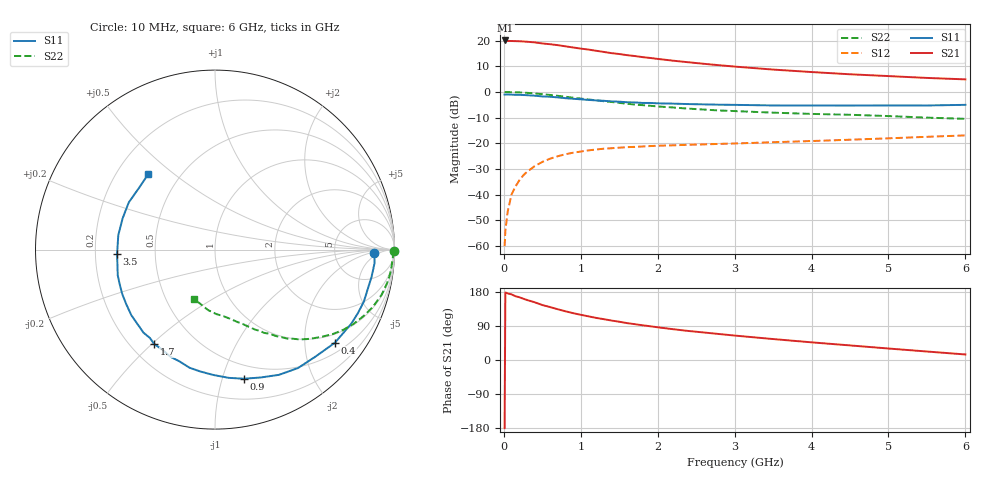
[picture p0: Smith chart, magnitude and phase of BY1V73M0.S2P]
! SIEMENS Small Signal Semiconductors
! BFY420
! Si NPN RF SIEGET Grounded Emitter Transistor in MICRO-X
! VCE = 1.75 V  IC = 3 mA
! Common Emitter S-Parameters:  October  1996
# GHz  S  MA  R  50
!  f  S11  S21  S12  S22
! GHz  MAG  ANG  MAG  ANG  MAG  ANG  MAG  ANG
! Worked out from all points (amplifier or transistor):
!   36 points, 10 MHz to 6 GHz, reference 50 ohm
!   highest |S21| = 20.0 dB at 20 MHz (marker M1)
!   |S21| within 3 dB of that: start of sweep to 962 MHz
!   unconditionally stable (mu >= 1): 3.603 GHz to end of sweep
!   at 250 MHz: K = 0.07, MSG = 26.1 dB, |S12| = -32.5 dB
!   at 1.4 GHz: K = 0.39, MSG = 18.5 dB, |S12| = -21.9 dB
!   at 6 GHz: K = 1.20, MAG = 8.2 dB, |S12| = -16.9 dB
!   S11 on the Smith chart (normalised r, x): 10 MHz: 16, -3; 400 MHz: 0.75, -2.74; 900 MHz: 0.37, -1.18; 1.7 GHz: 0.29, -0.51; 3.5 GHz: 0.29, -0.02; 6 GHz: 0.33, +0.41
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0.01  0.8887 -1.3  9.978 -179.8  0.001 111.1  0.9949 -0.5
0.02  0.8891 -2.0  10.04 178.2  0.002 96.4  0.992 -1.0
0.05  0.8923 -4.8  9.824 175.8  0.0047 90.2  0.9919 -2.5
0.1  0.8855 -9.8  9.789 173.1  0.0101 86.8  0.9884 -5.2
0.15  0.879 -14.4  9.742 168.4  0.0144 80.3  0.9851 -7.8
0.2  0.8785 -19.3  9.678 165.7  0.0189 79.5  0.9796 -10.2
0.3  0.8643 -28.5  9.48 158.4  0.0279 73.9  0.9616 -15.2
0.4  0.846 -37.8  9.211 152.4  0.0359 68.8  0.9355 -20.0
0.5  0.8184 -46.5  8.774 145.1  0.0435 64.6  0.9061 -24.2
0.7  0.7837 -62.9  8.139 134.0  0.0561 56.6  0.8413 -32.2
0.9  0.737 -77.4  7.324 123.6  0.0658 49.1  0.7734 -38.7
1.1  0.6991 -90.5  6.671 115.2  0.073 44.1  0.714 -44.3
1.2  0.6845 -96.7  6.322 111.1  0.076 41.6  0.6863 -46.8
1.4  0.6538 -107.5  5.681 104.1  0.0804 37.5  0.6377 -51.0
1.7  0.6255 -122.9  5.001 94.6  0.0854 33.2  0.5683 -56.3
2  0.6008 -135.0  4.395 86.3  0.0899 29.7  0.5224 -60.6
2.2  0.5924 -141.9  4.055 81.3  0.0916 27.9  0.4985 -63.4
2.8  0.565 -159.9  3.309 68.5  0.0976 24.7  0.4361 -70.4
3.5  0.5461 -177.6  2.724 55.3  0.1052 22.5  0.3955 -77.5
4.5  0.5433 161.1  2.206 38.5  0.1176 19.6  0.3595 -88.7
5.5  0.5456 140.6  1.873 22.4  0.134 16.4  0.3164 -103.7
6  0.5612 131.6  1.756 14.6  0.1429 14.2  0.2999 -112.7
